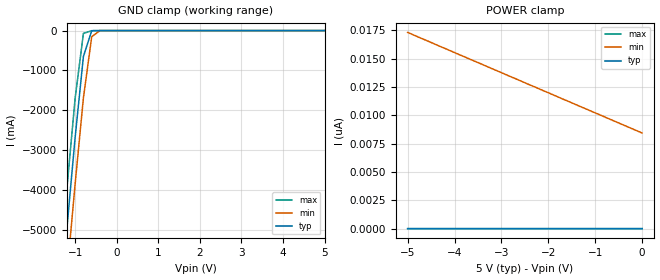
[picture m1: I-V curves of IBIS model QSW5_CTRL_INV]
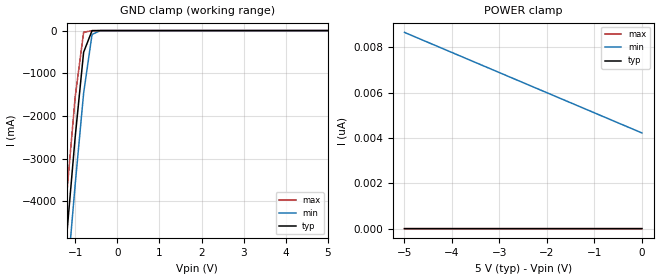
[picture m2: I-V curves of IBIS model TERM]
| I/O Buffer Information Specification (IBIS) Version 3.2 (August 20, 1999)
| IBIS is a standard for electronic behavioral specifications of integrated
| circuit input/output analog characteristics.
[IBIS Ver]   3.2
[File Name]   qs32x384.ibs
[File Rev]   2.0
[Date]   Wednesday, June 9, 2004
[Source]   Integrated Device Technology, Inc.
[Notes]   1.Temperatures: typ=25C, min=-40C, max=100C
[Disclaimer]
Integrated Device Technology, Inc. ("IDT") hereby grants the user of this
IBIS model ("User") a non-exclusive, nontransferable license to use this
IBIS model under the following terms: The User is granted this license only
to use the IBIS model for demonstration purposes only and is not granted
rights to sell, copy (except as needed to run the IBIS model), rent, lease
or sub-license (except for demonstration) the IBIS model in whole or in
part, or in modified form to anyone. The User may modify the IBIS model to
suit its specific applications, but  rights to derivative works and such
modifications shall belong to IDT.
THIS IBIS MODEL IS PROVIDED ON AN AS IS" BASIS AND IDT  MAKES ABSOLUTELY NO
WARRANTY WITH RESPECT TO THE INFORMATION CONTAINED HEREIN.  IDT DISCLAIMS
AND USER WAIVES ALL WARRANTIES, EXPRESS AND IMPLIED, INCLUDING WARRANTIES OF
MERCHANTABILITY AND FITNESS FOR A PARTICULAR PURPOSE.  THE ENTIRE RISK AS TO
QUALITY AND PERFORMANCE IS WITH THE USER  ACCORDINGLY, IN NO EVENT SHALL IDT
BE LIABLE FOR ANY DIRECT OR INDIRECT DAMAGES, WHETHER IN CONTRACT OR TORT,
INCLUDING ANY LOST PROFITS OR OTHER INCIDENTAL, CONSEQUENTIAL, EXEMPLARY, OR
PUNITIVE DAMAGES ARISING OUT OF THE USE OR APPLICATION OF THE  IBIS MODEL,
WHETHER OR NOT IDT HAD NOTICE OF SUCH DAMAGES.
IDT reserves the right to make changes without notice to any product herein
to improve reliability, function, or design. IDT does not convey any license
under patent rights or any other intellectual property rights, including
those of third parties. IDT is not obligated to provide maintenance or
support for the licensed IBIS model.
This model is for High-Speed CMOS 10-Bit Bus Switch.
[Copyright]
Copyright 2002, Integrated Device Technology, Inc. All rights reserved.
|   Component QS32X384
[Component]   QS32X384
[Manufacturer]   Integrated Device Technology
[Package]
|Following package parameters are for QVSOP 48 lead package
| variable   typ   min   max
R_pkg   0.01   0.01   0.01
L_pkg   2.50nH   2.50nH   2.50nH
C_pkg   0.40pF   0.40pF   0.40pF
[Pin]  signal_name   model_name   R_pin   L_pin   C_pin
1   _BEA_   QSW5_CTRL_INV
2   B0   TERM
3   A0   TERM
4   A1   TERM
5   B1   TERM
6   B2   TERM
7   A2   TERM
8   A3   TERM
9   B3   TERM
10   B4   TERM
11   A4   TERM
12   GND   GND
13   _BEC_   QSW5_CTRL_INV
14   B5   TERM
15   A5   TERM
16   A6   TERM
17   B6   TERM
18   B7   TERM
18   A7   TERM
20   A8   TERM
21   B8   TERM
22   B9   TERM
23   A9   TERM
24   GND   GND
25   _BED_   QSW5_CTRL_INV
26   A10   TERM
27   B10   TERM
28   B11   TERM
29   A11   TERM
30   A12   TERM
31   B12   TERM
32   B13   TERM
33   A13   TERM
34   A14   TERM
35   B14   TERM
36   VCC   POWER
37   _BEB_   QSW5_CTRL_INV
38   A15   TERM
39   B15   TERM
40   B16   TERM
41   A16   TERM
42   A17   TERM
43   B17   TERM
44   B18   TERM
45   A18   TERM
46   A19   TERM
47   B19   TERM
48   VCC   POWER
[Series Switch Groups]
|Function Group States
On A /
On B /
On C /
On D /
On A B /
On A B C /
On A B C D /
Off A /
Off B /
Off C /
Off D /
Off A B /
Off A B C /
Off A B C D /
[Series Pin Mapping]   pin_2   model_name   function_table_group
3   2   QSW5_SW   A
4   5   QSW5_SW   A
7   6   QSW5_SW   A
8   9   QSW5_SW   A
11   10   QSW5_SW   A
15   14   QSW5_SW   B
16   17   QSW5_SW   B
19   18   QSW5_SW   B
20   21   QSW5_SW   B
23   22   QSW5_SW   B
26   27   QSW5_SW   C
29   28   QSW5_SW   C
30   31   QSW5_SW   C
33   32   QSW5_SW   C
34   35   QSW5_SW   C
38   39   QSW5_SW   D
41   40   QSW5_SW   D
42   43   QSW5_SW   D
45   44   QSW5_SW   D
46   47   QSW5_SW   D
|   Model QSW5_SW
[Model]   QSW5_SW
Model_type   Series_switch
C_comp   0.0pF   0.0pF   0.0pf
[Temperature Range]   25.00   100.00   -40.00
[Voltage Range]   5.00V   4.75V   5.25V
[On]
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[Off]
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| Models and submodels in the file (3): QSW5_CTRL_INV (Input), TERM (Terminator), QSW5_SW (Series_switch)
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|   Model QSW5_CTRL_INV
[Model]   QSW5_CTRL_INV
Model_type   Input
Vinl =  0.80000V
Vinh =  2.00000V
C_comp   4.20000pF   4.20000pF   4.20000pF
[Temperature Range]   25.00000   100.00000   -40.00000
[Voltage Range]   5.00000V   4.75000V   5.25000V
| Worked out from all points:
|   GND clamp passes 1 mA (typ) near -0.48 V on its own axis
[GND_clamp]
| voltage   I(typ)   I(min)   I(max)
-5V       -51.74A    -52.8A     -50.85A
-1.4V     -7.368A    -8.538A    -6.375A
-1.2V     -4.993A    -6.169A    -3.993A
-1V       -2.692A    -3.858A    -1.708A
-800mV    -650.1mA   -1.689A    -70.61mA
-600mV    -2.541mA   -153.7mA   -3.31mA
-400mV    -3.914uA   -449.3uA   -30.03uA
5V        2.373pA    8.883nA    568.4fA
[POWER_clamp]
| voltage   I(typ)   I(min)   I(max)
-5V       3.268pA    17.31nA    739fA
-3.9V     3.055pA    15.35nA    710.5fA
-3.5V     2.998pA    14.65nA    682.1fA
0V        2.373pA    8.439nA    568.4fA
|   Model TERM
[Model]   TERM
Model_type   Terminator
Vinl =  0.80000V
Vinh =  2.00000V
C_comp   5.70000pF   5.70000pF   5.70000pF
[Temperature Range]   25.00000   100.00000   -40.00000
[Voltage Range]   5.00000V   4.75000V   5.25000V
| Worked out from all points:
|   GND clamp passes 1 mA (typ) near -0.55 V on its own axis
[GND_clamp]
| voltage   I(typ)   I(min)   I(max)
-5V       -51.52A    -52.53A    -50.68A
-1.4V     -7.155A    -8.273A    -6.207A
-1.2V     -4.784A    -5.908A    -3.829A
-1V       -2.494A    -3.606A    -1.556A
-800mV    -507mA     -1.468A    -40.58mA
-600mV    -1.329mA   -90.06mA   -2.011mA
-400mV    -2.283uA   -225uA     -18.42uA
5V        1.357pA    4.443nA    334fA
[POWER_clamp]
| voltage   I(typ)   I(min)   I(max)
-5V       1.805pA    8.655nA    397.9fA
-4.8V     1.776pA    8.477nA    426.3fA
-600mV    1.407pA    4.753nA    355.3fA
0V        1.357pA    4.222nA    326.8fA
